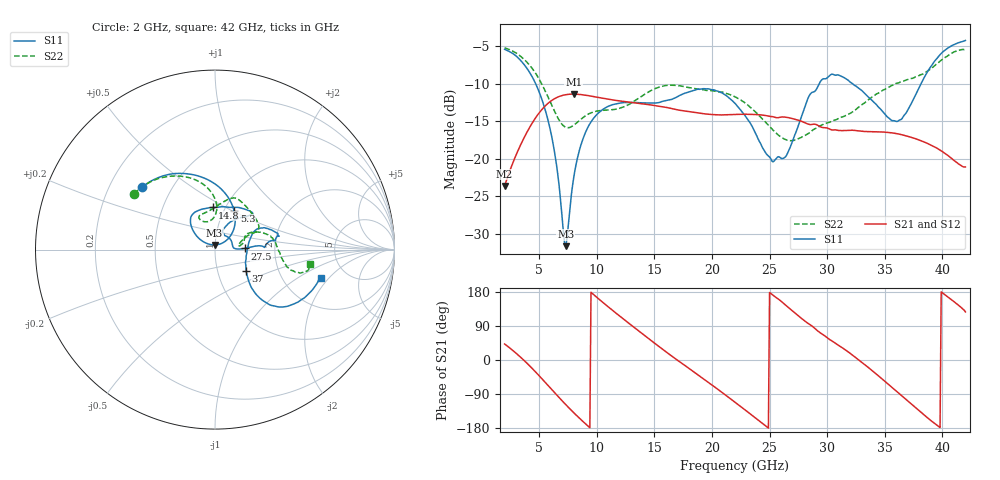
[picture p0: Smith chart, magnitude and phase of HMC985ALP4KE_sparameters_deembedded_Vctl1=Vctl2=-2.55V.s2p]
!s2p File: Measurements: S11, S21, S12, S22
# GHz S dB R 50.0
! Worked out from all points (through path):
!   401 points, 2 GHz to 42 GHz, reference 50 ohm
!   highest |S21| = -11.39 dB at 8 GHz (marker M1); lowest = -23.6 dB at 2 GHz (marker M2)
!   lowest |S11| = -31.6 dB at 7.3 GHz (marker M3), VSWR 1.05, Z = 49.7 + j2.59 ohm
!   |S11| at or under -10 dB: 4.693 GHz to 29.32 GHz (24.62 GHz wide, 145 % of centre); 32.2 GHz to 38.15 GHz (5.954 GHz wide, 16.9 % of centre)
!   |S22| runs from -17.6 to -5.2 dB; largest |S21 - S12| = 0.00027
!   S11 on the Smith chart (normalised r, x): 2 GHz: 0.34, +0.33; 5.3 GHz: 1.12, +0.51; 14.8 GHz: 0.87, +0.43; 27.5 GHz: 1.40, +0.02; 37 GHz: 1.37, -0.34; 42 GHz: 3.26, -1.66
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2  -5.42 139.3  -23.63 42.3  -23.64 42.3  -5.22 145.5
3.6  -7.28 105.7  -17.48 1.4  -17.48 1.4  -6.64 118.3
5.3  -12.38 63.6  -13.33 -51.5  -13.33 -51.5  -10.26 92.3
6.3  -18.79 41.6  -12.03 -84.9  -12.04 -84.9  -13.55 88.0
7.3  -31.64 95.5  -11.47 -117.5  -11.47 -117.5  -15.81 100.6
8  -22.50 145.7  -11.39 -139.1  -11.39 -139.1  -15.53 111.4
8.7  -17.80 143.3  -11.47 -159.4  -11.47 -159.4  -14.65 116.4
10  -14.12 133.5  -11.80 165.4  -11.80 165.4  -13.65 114.7
11.9  -12.62 121.6  -12.28 118.1  -12.29 118.1  -13.33 100.7
14.8  -12.58 93.2  -12.86 49.4  -12.86 49.4  -10.85 76.0
15.4  -12.51 85.9  -13.01 35.6  -13.02 35.6  -10.47 72.6
19.2  -10.68 45.5  -13.99 -48.3  -14.00 -48.3  -10.82 43.8
22  -12.62 50.2  -14.10 -111.5  -14.11 -111.4  -11.74 23.8
25.3  -20.41 54.9  -14.40 171.0  -14.41 171.0  -16.21 17.8
26.4  -19.71 5.7  -14.46 144.6  -14.47 144.6  -17.45 11.6
27.5  -15.56 2.3  -14.87 116.6  -14.87 116.5  -17.33 8.5
28.7  -11.15 2.5  -15.42 89.2  -15.43 89.2  -16.24 11.5
31.1  -8.92 14.9  -16.24 36.6  -16.25 36.6  -14.56 24.7
35.4  -14.63 6.4  -16.51 -66.4  -16.51 -66.5  -10.44 16.5
37  -13.51 -34.7  -17.01 -108.4  -17.02 -108.4  -9.45 7.5
39.7  -6.31 -41.4  -18.74 -175.9  -18.75 -176.0  -7.15 -15.1
42  -4.25 -15.0  -21.09 126.9  -21.09 126.9  -5.41 -8.9
